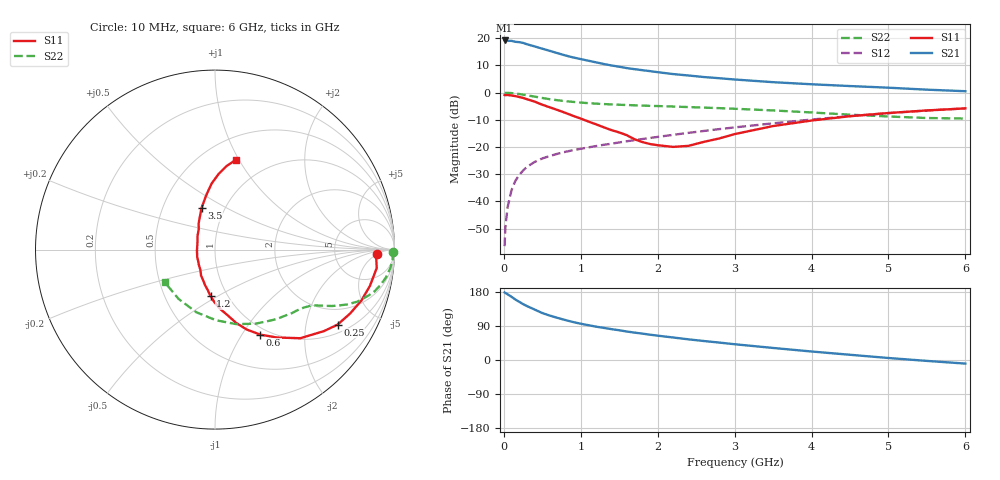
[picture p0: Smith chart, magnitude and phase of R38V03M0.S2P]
! SIEMENS Small Signal Semiconductors
! BFR181
! Si NPN RF Bipolar Junction Transistor in SOT23
! VCE = 8 V  IC = 3 mA
! Common Emitter S-Parameters:  May  1996
# GHz  S  MA  R  50
!  f  S11  S21  S12  S22
! GHz  MAG  ANG  MAG  ANG  MAG  ANG  MAG  ANG
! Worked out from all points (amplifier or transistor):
!   36 points, 10 MHz to 6 GHz, reference 50 ohm
!   highest |S21| = 19.2 dB at 10 MHz (marker M1)
!   |S21| within 3 dB of that: start of sweep to 495.8 MHz
!   unconditionally stable (mu >= 1): 1.426 GHz to 3.278 GHz
!   at 250 MHz: K = 0.29, MSG = 23.5 dB, |S12| = -28.7 dB
!   at 1.4 GHz: K = 1.00, MSG = 14.4 dB, |S12| = -18.8 dB
!   at 6 GHz: K = 0.86, MSG = 3.2 dB, |S12| = -5.8 dB
!   lowest NFmin = 1.40 dB at 450 MHz
!   S11 on the Smith chart (normalised r, x): 10 MHz: 19, -5; 250 MHz: 1.30, -3.03; 600 MHz: 0.91, -1.21; 1.2 GHz: 0.83, -0.46; 3.5 GHz: 0.78, +0.38; 6 GHz: 0.72, +0.97
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0.01  0.9049 -1.5  9.127 178.2  0.0015 89.4  0.9942 -0.7
0.02  0.8988 -2.5  8.877 176.8  0.0034 90.8  0.9897 -1.3
0.05  0.9068 -6.5  8.975 173.2  0.008 88.1  0.9914 -3.2
0.1  0.8866 -13.2  8.973 166.8  0.0161 82.3  0.9809 -6.3
0.15  0.8635 -19.2  8.62 159.6  0.0239 78.0  0.9641 -9.4
0.2  0.8323 -25.4  8.494 153.6  0.0307 75.1  0.9437 -12.0
0.25  0.8006 -31.5  8.225 147.5  0.0369 72.4  0.9193 -14.6
0.3  0.7581 -36.8  7.777 142.3  0.0431 70.2  0.8934 -16.6
0.4  0.6852 -46.1  7.093 133.2  0.0531 66.2  0.8462 -20.0
0.5  0.5995 -54.8  6.435 123.9  0.0616 63.2  0.7983 -22.5
0.6  0.5365 -62.0  5.86 117.0  0.0686 61.1  0.7565 -24.3
0.8  0.4252 -73.9  4.834 105.4  0.0815 58.7  0.6978 -26.7
0.9  0.3745 -78.9  4.45 100.2  0.0876 58.3  0.6765 -27.5
1.1  0.2939 -90.5  3.864 91.8  0.0984 58.6  0.6406 -29.0
1.2  0.2609 -95.4  3.608 87.9  0.1042 58.5  0.6275 -29.8
1.6  0.1646 -118.1  2.83 75.1  0.1277 58.9  0.5923 -33.0
2.2  0.1006 -176.9  2.198 59.4  0.1674 58.9  0.5561 -39.5
2.6  0.1244 141.4  1.939 50.1  0.1974 57.9  0.5307 -44.8
3.5  0.2432 108.0  1.559 31.8  0.2728 53.2  0.4711 -61.1
4.5  0.3687 92.9  1.323 13.8  0.37 44.2  0.3936 -89.2
5.5  0.4713 82.0  1.135 -2.4  0.4684 32.2  0.3417 -126.4
6  0.5136 76.8  1.063 -9.5  0.5146 25.2  0.3338 -147.0
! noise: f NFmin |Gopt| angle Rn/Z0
0.45  1.4  0.56  17  0.36
0.9  1.5  0.45  35  0.34
1.8  1.85  0.25  82  0.36
